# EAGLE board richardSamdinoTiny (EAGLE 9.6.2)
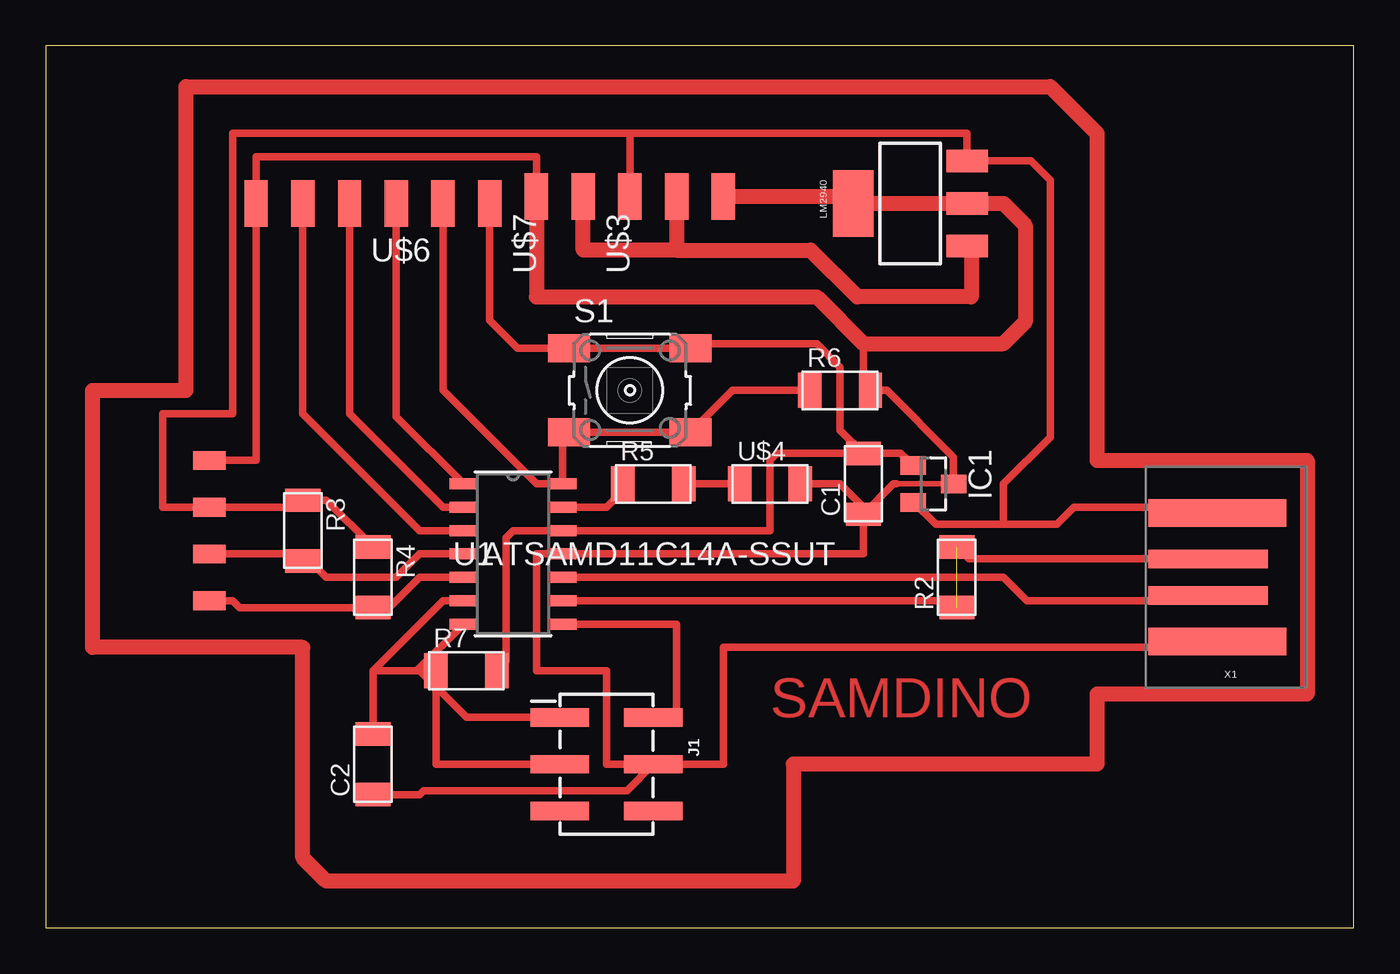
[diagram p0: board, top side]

Size 71.1 x 47.93 mm. Coordinates in mm from the lower left corner, seen from the top.
Outline: 0,0 71.1,0 71.1,47.93 0,47.93 0,0
Copper layers (1*16): Top 0.035mm / dielectric 1.5mm / Bottom 0.035mm
Design rules "default *": minimum track width 16mil, minimum drill 0.35mm, track to track 16mil, track to pad 16mil, pad to pad 16mil, via to via 16mil, smd to smd 6mil, copper to edge 40mil, drill to drill 16mil, minimum pad ring 10mil, minimum via ring 8mil, stop-mask expansion 4mil, vias tented up to drill 0mil, thermal gap 10mil

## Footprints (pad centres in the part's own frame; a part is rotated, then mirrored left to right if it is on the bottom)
C1206FAB = smd 1.27 x 1.905: 1 -1.651,0; 2 1.651,0
SOT23 = smd 1 x 1.4: 1 -1.001,-1.1; 2 1.014,-1.1; 3 0,1.1
2X3_SMT_POSTS = smd 1 x 3.17: 1 -2.54,-2.54; 2 -2.54,2.54; 3 0,-2.54; 4 0,2.54; 5 2.54,-2.54; 6 2.54,2.54
1X04SMD/90 = smd 1.016 x 1.778: 1 -1.27,-5.08; 2 1.27,-5.08; 3 3.81,-5.08; 4 6.35,-5.08
SOT223 = smd 1.219 x 2.235: 1 -2.311,-3.099; 2 0,-3.099; 3 2.311,-3.099 | smd 3.6 x 2.2: 4 0,3.099
R1206FAB = smd 1.27 x 1.905: 1 -1.651,0; 2 1.651,0
6MM_SWITCH = smd 2.286 x 1.524: 1 -3.302,2.286; 2 3.302,2.286; 3 -3.302,-2.286; 4 3.302,-2.286
SOIC14_SL_MCH = smd 1.5 x 0.6: 1 -2.7,3.81; 2 -2.7,2.54; 3 -2.7,1.27; 4 -2.7,0; 5 -2.7,-1.27; 6 -2.7,-2.54; 7 -2.7,-3.81; 8 2.7,-3.81; 9 2.7,-2.54; 10 2.7,-1.27; 11 2.7,0; 12 2.7,1.27; 13 2.7,2.54; 14 2.7,3.81
SPDTSWITCH = smd 2.54 x 1.27: 1 0.38,2.54; 2 0.38,0; 3 0.38,-2.54
LED1206FAB = smd 1.27 x 1.905: 1 -1.651,0; 2 1.651,0
1X06SMD = smd 2.54 x 1.27: 1 0,6.35; 2 0,3.81; 3 0,1.27; 4 0,-1.27; 5 0,-3.81; 6 0,-6.35
USB-A-PCB = smd 7.5 x 1.5: 5V -0.2,-3.5; GND -0.2,3.5 | smd 6.5 x 1: USB_M 0.3,-1; USB_P 0.3,1

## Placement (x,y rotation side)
C1  1uF  [C1206FAB]  44.45,24.13 90 top
C2  1uF  [C1206FAB]  17.78,8.89 90 top
IC1  [SOT23]  48.26,24.13 270 top
J1  [2X3_SMT_POSTS]  30.48,8.89 270 top
JP3  [1X04SMD/90]  13.97,24.13 270 top
LM2940  VR_REGULATOR_SOT223  [SOT223]  46.99,39.37 90 top
R2  0  [R1206FAB]  49.53,19.05 90 top
R3  4.99K  [R1206FAB]  13.97,21.59 270 top
R4  4.99K  [R1206FAB]  17.78,19.05 270 top
R5  1K  [R1206FAB]  33.02,24.13 0 top
R6  470  [R1206FAB]  43.18,29.21 0 top
R7  10K  [R1206FAB]  22.86,13.97 0 top
S1  [6MM_SWITCH]  31.75,29.21 0 top
U1  ATSAMD11C14A-SSUT  [SOIC14_SL_MCH]  25.4,20.32 0 top
U$3  SPDTSWITCH  [SPDTSWITCH]  34.29,39.37 90 top
U$4  LEDFAB1206  [LED1206FAB]  39.37,24.13 0 top
U$6  CONN_06_FTDI-SMD-HEADER  [1X06SMD]  17.78,39.37 90 top
U$7  SPDTSWITCH  [SPDTSWITCH]  29.21,39.37 90 top
X1  CONN_USBPCB  [USB-A-PCB]  63.5,19.05 180 top

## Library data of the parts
C1 C2 IC1 LM2940 R2-R7 S1 U$3 U$4 U$6 U$7 X1 = fab
J1 = fab; PROD_ID: CONN-11415
JP3 = pinhead-2
U1 = samd11c; BUILT_BY: EMA_Molly; COPYRIGHT: Copyright (C) 2018 Accelerated Designs. All rights reserved; MANUFACTURER_PART_NUMBER: ATSAMD11C14A-SSUT; SOURCELIBRARY: Microchip_2019-08-23_25; VENDOR: Microchip

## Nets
2: R5.1 U1.13
4: R6.1 S1.3 S1.4 U1.14 U$6.5
5: U1.1 U$6.4
5V: IC1.2 JP3.2 LM2940.3 R3.1 R4.1 U$3.1 U$7.3 X1.5V
8: U1.2 U$6.3
9: U1.3 U$6.2
24-: R2.1 R2.2 U1.9 X1.USB_M
25+: U1.10 X1.USB_P
CLK: J1.1 U1.7
DIO: J1.2 U1.8
GND: C1.1 C2.1 IC1.3 J1.4 JP3.1 LM2940.2 LM2940.4 R6.2 U1.11 U$3.3 U$4.2 U$6.1 U$7.1 X1.GND
N$5: R5.2 U$4.1
RST: C2.2 J1.3 R7.1 U1.6
SCL: JP3.4 R4.2 U1.5
SDA: JP3.3 R3.2 U1.4
VD0: LM2940.1 U$3.2 U$7.2
VDD: C1.2 IC1.1 R7.2 S1.1 S1.2 U1.12 U$6.6

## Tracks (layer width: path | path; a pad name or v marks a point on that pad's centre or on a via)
2
  Top 0.406: U1.13 30.48,22.86 31.37,23.75 R5.1
4
  Top 0.406: S1.3 28.1,26.58 U1.14 26.67,24.13 21.59,29.21 U$6.5 | S1.3 28.7,26.67 | S1.3 28.96,26.92 | S1.3 S1.4 37.34,29.21 R6.1
5
  Top 0.406: U1.1 19.05,27.78 U$6.4
5V
  Top 0.406: X1.5V 63.39,22.86 55.88,22.86 54.97,21.95 52.07,21.95 | IC1.2 48.39,21.95 52.07,21.95 | 52.07,21.95 52.07,24.13 54.61,26.67 54.61,40.64 53.57,41.68 LM2940.3 50.09,43.18 31.75,43.18 | 31.75,43.18 U$7.3 | R4.1 15.24,23.24 R3.1 13.59,22.86 JP3.2 6.35,22.86 6.35,27.94 10.16,27.94 10.16,43.18 31.75,43.18
8
  Top 0.406: U1.2 21.59,22.86 16.51,27.94 U$6.3
9
  Top 0.406: U1.3 20.32,21.59 13.97,27.94 U$6.2
24-  (1 unrouted)
  Top 0.406: 27.94,17.78 U1.9 49.15,17.78 R2.1 | R2.2 50.18,20.05 X1.USB_M
25+
  Top 0.406: U1.10 52.07,19.05 53.34,17.78 62.93,17.78 X1.USB_P
CLK
  Top 0.406: 22.7,16.35 U1.7 20.24,14.05 22.86,11.43 J1.1
DIO
  Top 0.406: U1.8 34.29,16.51 34.29,11.43 J1.2
GND
  Top 0.305: 46.25,24.12 IC1.3
  Top 0.406: X1.GND 63.39,15.24 36.83,15.24 36.83,8.89 J1.4 | C1.1 44.45,20.32 U1.11 26.67,20.32 26.67,13.97 30.48,13.97 30.48,8.89 J1.4 | C1.1 44.45,22.86 43.18,24.13 U$4.2 | C1.1 46.09,24.12 46.25,24.12 | 49.53,24.3 IC1.3 49.35,25.58 45.72,29.21 R6.2 44.45,29.59 44.45,31.75 | U$7.1 26.67,41.91 11.43,41.91 U$6.1 11.43,25.4 JP3.1 | C2.1 20.32,7.24 20.54,7.46 31.59,7.46 J1.4
  Top 0.813: U$3.3 43.89,39.75 LM2940.4 LM2940.2 52.07,39.37 53.26,38.18 53.26,32.94 52.07,31.75 44.45,31.75 41.91,34.29 26.67,34.29 U$7.1
N$1
  Top 0.813: 7.62,45.72 54.61,45.72 57.15,43.18 57.15,25.4 68.58,25.4 68.58,12.7 57.15,12.7 57.15,8.89 40.64,8.89 40.64,2.54 15.24,2.54 13.97,3.81 13.97,15.24 2.54,15.24 2.54,29.21 7.62,29.21 7.62,45.72
N$5
  Top 0.406: R5.2 U$4.1
RST
  Top 0.406: U1.6 21.59,17.78 17.78,13.97 | 17.78,13.97 C2.2 | 17.78,13.97 R7.1 21.21,8.89 J1.3
SCL
  Top 0.406: U1.5 20.32,19.05 18.67,17.4 R4.2 10.54,17.4 10.16,17.78 JP3.4
SDA
  Top 0.406: U1.4 20.32,20.32 19.05,19.05 15.24,19.05 14.35,19.94 R3.2 13.59,20.32 JP3.3
VD0
  Top 0.813: U$3.2 34.29,36.83 | 34.29,36.83 41.58,36.83 44.12,34.29 50.32,34.29 50.32,36.83 LM2940.1 | 34.29,36.83 29.21,36.83 U$7.2
VDD
  Top 0.406: 46.84,25.4 IC1.1 46.46,25.78 C1.2 | C1.2 39.75,25.78 39.37,25.4 39.37,21.59 U1.12 25.4,21.59 25.02,21.21 25.02,14.48 R7.2 | C1.2 43.18,27.05 43.18,30.48 41.91,31.75 35.31,31.75 S1.2 S1.1 25.65,31.5 24.13,33.02 U$6.6

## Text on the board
Top: SAMDINO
